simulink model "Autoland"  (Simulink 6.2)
settings: Solver=ode45  StartTime=0.0  StopTime=100  RelTol=1e-3
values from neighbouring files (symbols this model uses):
  Agu = [    [guidance.m]
  Ave = [    [pitch_vehi3.m]    (also in Siso_Anal.m; vehi_latan2.m; vehi_ldes.m)
  Bgu = [    [guidance.m]
  Bve = [    [pitch_vehi3.m]    (also in Siso_Anal.m; vehi_latan2.m; vehi_ldes.m)
  Cgu = [    [guidance.m]
  Cve = [    [pitch_vehi3.m]    (also in Siso_Anal.m; vehi_latan2.m; vehi_ldes.m)
  Dgu = [    [guidance.m]
  Dve = [    [pitch_vehi3.m]    (also in Siso_Anal.m; vehi_latan2.m; vehi_ldes.m)
  x0 = [0.1, -0.08, 0.18, 9000, 50, zeros(1,8)]    [run.m]
undefined symbols (not defined in the file or in its folder): sigbuilder_block

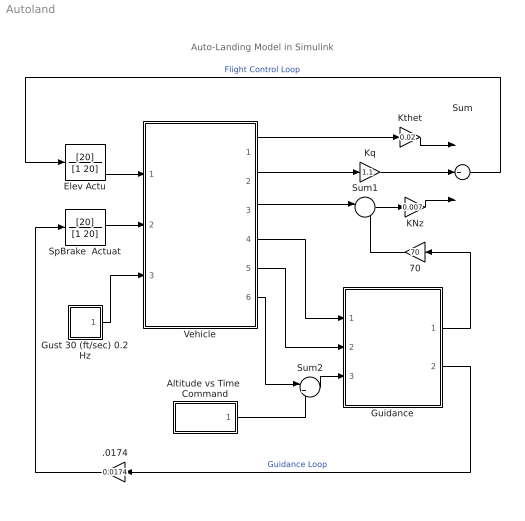
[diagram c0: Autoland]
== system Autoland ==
  note: Auto-Landing Model in Simulink
  .0174 : Gain  Orientation=left  Gain=0.0174
  70 : Gain  Orientation=left  Gain=70
  Altitude vs Time  Command : Subsystem  Tag=STV Subsys  LoadFcn=sigbuilder_block('load');  StartFcn=sigbuilder_block('start');  StopFcn=sigbuilder_block('stop');  ClipboardFcn=sigbuilder_block('clipboard');
  Elev Actu : TransferFcn  Numerator=[20]  Denominator=[1 20]
  Guidance : Subsystem
  Gust 30 (ft/sec) 0.2 Hz : Subsystem
  KNz : Gain  Gain=0.007
  Kq : Gain  Gain=1.1
  Kthet : Gain  Gain=0.02
  SpBrake  Actuat : TransferFcn  Numerator=[20]  Denominator=[1 20]
  Sum : Sum  Inputs=+++  OutScaling=2^-10
  Sum1 : Sum  Inputs=|-+
  Sum2 : Sum  Inputs=|+-
  Vehicle : Subsystem
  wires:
  Elev Actu/1 -> Vehicle/1(Elevon)
  SpBrake  Actuat/1 -> Vehicle/2(Sp_Brake)
  Kthet/1 -> Sum/1
  Vehicle/2(q) -> Kq/1
  Kq/1 -> Sum/2
  KNz/1 -> Sum/3
  Sum/1 -> Elev Actu/1  "Flight Control Loop"
  Vehicle/3(Acc_Z) -> Sum1/1
  Sum1/1 -> KNz/1
  Guidance/1(Nz-com) -> 70/1
  Guidance/2(SpBrak-com) -> .0174/1  "Guidance Loop"
  Sum2/1 -> Guidance/3(dH)
  Vehicle/6(dH) -> Sum2/1
  Vehicle/5(dH-dot) -> Guidance/2(H-dot)
  Vehicle/4(dV) -> Guidance/1(dV)
  70/1 -> Sum1/2
  .0174/1 -> SpBrake  Actuat/1
  Vehicle/1(theta) -> Kthet/1
  Gust 30 (ft/sec) 0.2 Hz/1(Gust) -> Vehicle/3(Gust)
  Altitude vs Time  Command/1(Signal 3) -> Sum2/2

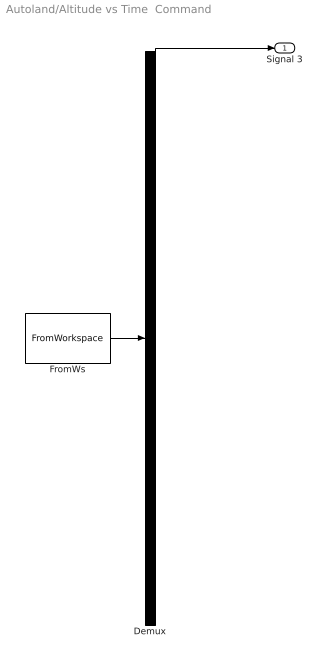
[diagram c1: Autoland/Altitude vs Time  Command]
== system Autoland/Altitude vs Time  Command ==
  Demux : Demux  Tag=STV Demux  Outputs=1
  FromWs : FromWorkspace  Tag=STV FromWs  VariableName=tuvar  SampleTime=0  SigBuilderData=DataTag0  VnvData=DataTag1
  Signal 3 : Outport  Tag=STV Outport
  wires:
  FromWs/1 -> Demux/1
  Demux/1 -> Signal 3/1

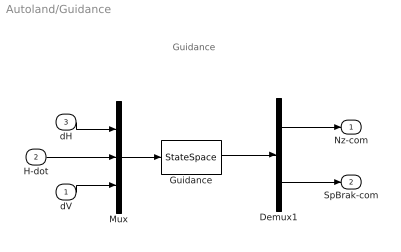
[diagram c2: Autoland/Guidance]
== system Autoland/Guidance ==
  note: Guidance
  dV : Inport  Port=1  LatchInput=off
  H-dot : Inport  Port=2  LatchInput=off
  dH : Inport  Port=3  LatchInput=off
  Demux1 : Demux  Outputs=2
  Guidance : StateSpace  A=Agu  B=Bgu  C=Cgu  D=Dgu
  Mux : Mux  Inputs=3
  Nz-com : Outport
  SpBrak-com : Outport  Port=2
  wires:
  dH/1 -> Mux/1
  H-dot/1 -> Mux/2
  dV/1 -> Mux/3
  Mux/1 -> Guidance/1
  Guidance/1 -> Demux1/1
  Demux1/2 -> SpBrak-com/1
  Demux1/1 -> Nz-com/1

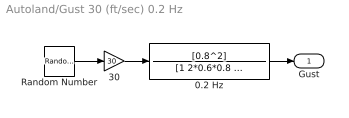
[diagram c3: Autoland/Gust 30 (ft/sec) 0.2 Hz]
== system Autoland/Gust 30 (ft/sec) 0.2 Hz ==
  0.2 Hz : TransferFcn  Numerator=[0.8^2]  Denominator="[1 2*0.6*0.8  0.8^2]"
  30 : Gain  Gain=30
  Random Number : RandomNumber  SampleTime=0
  Gust : Outport
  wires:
  30/1 -> 0.2 Hz/1
  Random Number/1 -> 30/1
  0.2 Hz/1 -> Gust/1

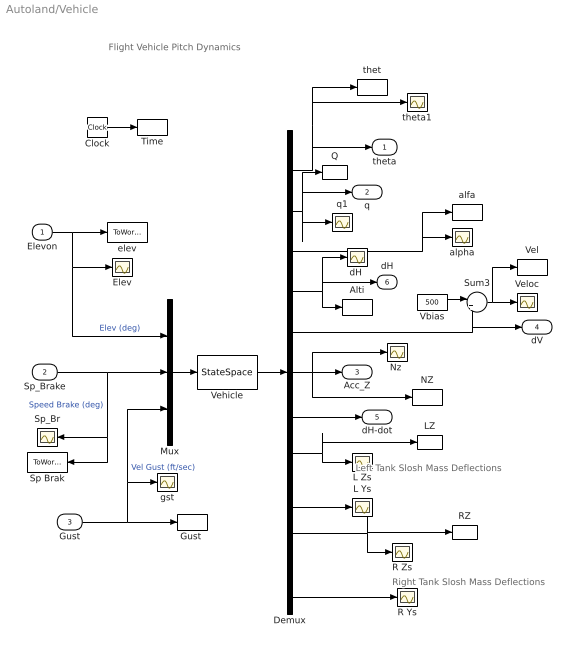
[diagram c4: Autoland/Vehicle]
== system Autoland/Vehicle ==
  note: Flight Vehicle Pitch Dynamics
  note: Right Tank Slosh Mass Deflections
  note: Left Tank Slosh Mass Deflections
  Elevon : Inport  Port=1  LatchInput=off
  Sp_Brake : Inport  Port=2  LatchInput=off
  Gust : Inport  Port=3  LatchInput=off
  Alti : ToWorkspace  VariableName=Alti  SampleTime=-1  SaveFormat=Array
  Clock : Clock
  Demux : Demux  Outputs=11
  Elev : Scope
  "Gust " : ToWorkspace  VariableName=Gust  SampleTime=-1  SaveFormat=Array
  L Ys : Scope
  L Zs : Scope
  LZ : ToWorkspace  VariableName=LZs  SampleTime=-1  SaveFormat=Array
  Mux : Mux  Inputs=3
  NZ : ToWorkspace  VariableName=Nz  SampleTime=-1  SaveFormat=Array
  "Nz " : Scope
  Q : ToWorkspace  VariableName=q  SampleTime=-1  SaveFormat=Array
  R Ys : Scope
  R Zs : Scope
  RZ : ToWorkspace  VariableName=RZs  SampleTime=-1  SaveFormat=Array
  Sp Brak : ToWorkspace  VariableName=SpBrake  SampleTime=-1  SaveFormat=Array
  Sp_Br : Scope
  Sum3 : Sum  Inputs=|++
  Time : ToWorkspace  VariableName=time  SampleTime=-1  SaveFormat=Array
  Vbias : Constant  Value=500
  Vehicle : StateSpace  A=Ave  B=Bve  C=Cve  D=Dve  X0=x0
  Vel : ToWorkspace  VariableName=Vel  SampleTime=-1  SaveFormat=Array
  Veloc : Scope
  alfa : ToWorkspace  VariableName=alpha  SampleTime=-1  SaveFormat=Array
  alpha : Scope
  "dH " : Scope
  elev : ToWorkspace  VariableName=Elevon  SampleTime=-1  SaveFormat=Array
  gst : Scope
  q1 : Scope
  thet : ToWorkspace  VariableName=theta  SampleTime=-1  SaveFormat=Array
  theta1 : Scope
  theta : Outport
  q : Outport  Port=2
  Acc_Z : Outport  Port=3
  dV : Outport  Port=4
  dH-dot : Outport  Port=5
  dH : Outport  Port=6
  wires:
  Mux/1 -> Vehicle/1
  Demux/1 -> theta/1, theta1/1, thet/1
  Demux/2 -> q/1, Q/1, q1/1
  Demux/3 -> alpha/1, alfa/1
  Demux/4 -> dH/1, "dH "/1, Alti/1
  Demux/5 -> dV/1, Sum3/2
  Gust/1 -> "Gust "/1, Mux/3, gst/1  "Vel Gust (ft/sec)"
  Demux/6 -> Acc_Z/1, "Nz "/1, NZ/1
  Demux/7 -> dH-dot/1
  Elevon/1 -> elev/1, Mux/1, Elev/1  "Elev (deg)"
  Sp_Brake/1 -> Mux/2, Sp Brak/1, Sp_Br/1  "Speed Brake (deg)"
  Clock/1 -> Time/1
  Vbias/1 -> Sum3/1
  Sum3/1 -> Veloc/1, Vel/1
  Vehicle/1 -> Demux/1
  Demux/8 -> L Zs/1, LZ/1
  Demux/9 -> L Ys/1
  Demux/10 -> R Zs/1, RZ/1
  Demux/11 -> R Ys/1
